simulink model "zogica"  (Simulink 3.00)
settings: Solver=ode45  StartTime=0.0  StopTime=10  RelTol=1e-6

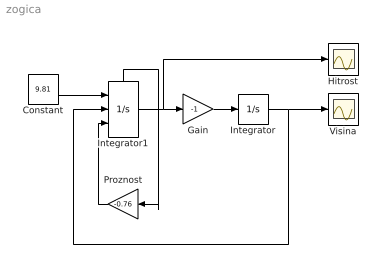
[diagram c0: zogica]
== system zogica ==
  Constant : Constant  Value=9.81
  Gain : Gain  Gain=-1  SaturateOnIntegerOverflow=on
  Hitrost : Scope
  Integrator : Integrator  ExternalReset=none  InitialConditionSource=internal  InitialCondition=10  LimitOutput=on  UpperSaturationLimit=inf  LowerSaturationLimit=0  ShowSaturationPort=off  ShowStatePort=off  AbsoluteTolerance=auto
  Integrator1 : Integrator  ExternalReset=falling  InitialConditionSource=external  InitialCondition=0  LimitOutput=off  UpperSaturationLimit=inf  LowerSaturationLimit=-inf  ShowSaturationPort=off  ShowStatePort=on  AbsoluteTolerance=auto
  Proznost : Gain  Orientation=left  Gain=-0.76  SaturateOnIntegerOverflow=on
  Visina : Scope
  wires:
  Integrator1/1 -> Gain/1, Hitrost/1
  Gain/1 -> Integrator/1
  Constant/1 -> Integrator1/1
  Integrator/1 -> Integrator1/2, Visina/1
  Proznost/1 -> Integrator1/3
  Integrator1/State -> Proznost/1
